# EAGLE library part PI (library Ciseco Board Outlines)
Ciseco Rasbperry Pi add on board outlines
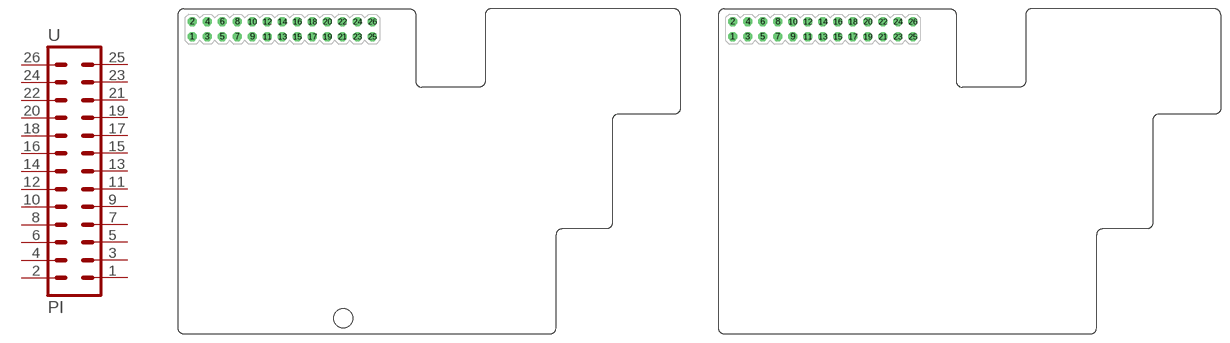
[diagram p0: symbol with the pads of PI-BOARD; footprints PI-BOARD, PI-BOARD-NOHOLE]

Designator prefix U

## PI  [PI-BOARD]
1  1  pas
2  2  pas
3  3  pas
4  4  pas
5  5  pas
6  6  pas
7  7  pas
8  8  pas
9  9  pas
10  10  pas
11  11  pas
12  12  pas
13  13  pas
14  14  pas
15  15  pas
16  16  pas
17  17  pas
18  18  pas
19  19  pas
20  20  pas
21  21  pas
22  22  pas
23  23  pas
24  24  pas
25  25  pas
26  26  pas

## PI-NOHOEL  [PI-BOARD-NOHOLE]
Pads as for PI-BOARD

## PI-REFRENCE  [PI-BOARD_REF]
Pads as for PI-BOARD

## PILARGER  [PI-HEADER-LARGEHOLES]
Pads as for PI-BOARD

## PI-REFRENCE-LOCK  [PI-BOARD-REF-LOCK]
Pads as for PI-BOARD

## PI-REFRENCE-LOCK-PASTE  [PI-BOARD-REF-LOCK-PASTE]
Pads as for PI-BOARD

## PI-HEADER  [PI-HEADER]
Pads as for PI-BOARD

## PI-HEADER-PIN-NUMBERS  [PI-HEADER-PIN]
Pads as for PI-BOARD

## PI-HEADER-PIN-NUMBERS-JAMLOCK  [PI-HEADER-PIN-JAMLOCK]
Pads as for PI-BOARD

## PI-HLE-CONNECTOR-ONLY  [HLE-113-02-F-DV-BE]
Pads as for PI-BOARD

## PI-HLE-BOTTOM  [HLE-113-02-F-DV-BE-BOTTOM]
Pads as for PI-BOARD

## Footprint PI-BOARD (pad centres in mm)
drill 1.016 octagon: 1 2.44,50.31; 2 2.44,52.85; 3 4.98,50.31; 4 4.98,52.85; 5 7.52,50.31; 6 7.52,52.85; 7 10.06,50.31; 8 10.06,52.85; 9 12.6,50.31; 10 12.6,52.85; 11 15.14,50.31; 12 15.14,52.85; 13 17.68,50.31; 14 17.68,52.85; 15 20.22,50.31; 16 20.22,52.85; 17 22.76,50.31; 18 22.76,52.85; 19 25.3,50.31; 20 25.3,52.85; 21 27.84,50.31; 22 27.84,52.85; 23 30.38,50.31; 24 30.38,52.85; 25 32.92,50.31; 26 32.92,52.85
hole 3.2 at 28.019,2.638

## Footprint PI-BOARD-NOHOLE (pad centres in mm)
drill 1.016 octagon: 1 2.44,50.31; 2 2.44,52.85; 3 4.98,50.31; 4 4.98,52.85; 5 7.52,50.31; 6 7.52,52.85; 7 10.06,50.31; 8 10.06,52.85; 9 12.6,50.31; 10 12.6,52.85; 11 15.14,50.31; 12 15.14,52.85; 13 17.68,50.31; 14 17.68,52.85; 15 20.22,50.31; 16 20.22,52.85; 17 22.76,50.31; 18 22.76,52.85; 19 25.3,50.31; 20 25.3,52.85; 21 27.84,50.31; 22 27.84,52.85; 23 30.38,50.31; 24 30.38,52.85; 25 32.92,50.31; 26 32.92,52.85

## Footprint PI-BOARD_REF (pad centres in mm)
drill 1.016 octagon: 1 2.44,50.31; 2 2.44,52.85; 3 4.98,50.31; 4 4.98,52.85; 5 7.52,50.31; 6 7.52,52.85; 7 10.06,50.31; 8 10.06,52.85; 9 12.6,50.31; 10 12.6,52.85; 11 15.14,50.31; 12 15.14,52.85; 13 17.68,50.31; 14 17.68,52.85; 15 20.22,50.31; 16 20.22,52.85; 17 22.76,50.31; 18 22.76,52.85; 19 25.3,50.31; 20 25.3,52.85; 21 27.84,50.31; 22 27.84,52.85; 23 30.38,50.31; 24 30.38,52.85; 25 32.92,50.31; 26 32.92,52.85

## Footprint PI-HEADER-LARGEHOLES (pad centres in mm)
drill 1.5 octagon: 1 2.44,2.05; 2 2.44,4.59; 3 4.98,2.05; 4 4.98,4.59; 5 7.52,2.05; 6 7.52,4.59; 7 10.06,2.05; 8 10.06,4.59; 9 12.6,2.05; 10 12.6,4.59; 11 15.14,2.05; 12 15.14,4.59; 13 17.68,2.05; 14 17.68,4.59; 15 20.22,2.05; 16 20.22,4.59; 17 22.76,2.05; 18 22.76,4.59; 19 25.3,2.05; 20 25.3,4.59; 21 27.84,2.05; 22 27.84,4.59; 23 30.38,2.05; 24 30.38,4.59; 25 32.92,2.05; 26 32.92,4.59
